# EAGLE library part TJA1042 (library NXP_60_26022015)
High-speed CAN transceiver with Standby mode The TJA1042 is a high-speed CAN transceiver that provides an interface between a Controller Area Network (CAN) protocol controller and the physical two-wire CAN bus. The transceiver is designed for high-speed (up to 1 Mbit/s) CAN applications in the automotive industry, providing the differential transmit and receive capability to (a microcontroller with) a CAN protocol controller. The TJA1042 belongs to the third generation of high-speed CAN transceivers from NXP Semiconductors, offering significant improvements over first- and second-generation devices such as the TJA1040. It offers improved ElectroMagnetic Compatibility (EMC) and ElectroStatic Discharge (ESD) performance, and also features: Ideal passive behavior to the CAN bus when the supply voltage is off A very low-current Standby mode with bus wake-up capability TJA1042T/3 and TJA1042TK/3 can be interfaced directly to microcontrollers with supply voltages from 3 V to 5 V These features make the TJA1042 an excellent choice for all types of HS-CAN networks, in nodes that require a low-power mode with wake-up capability via the CAN bus. AAL Eindhoven MK
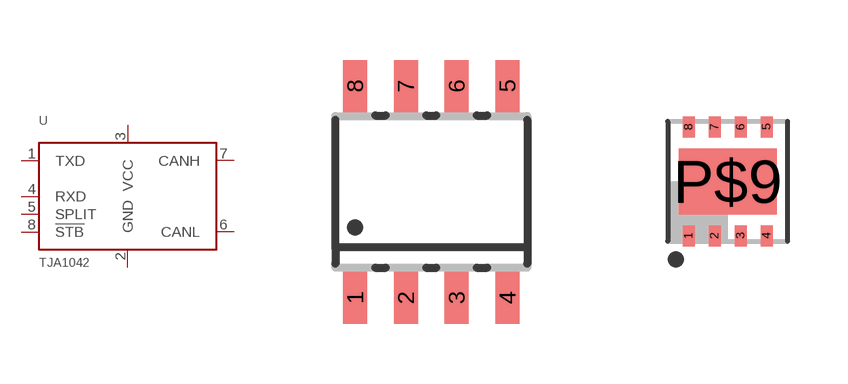
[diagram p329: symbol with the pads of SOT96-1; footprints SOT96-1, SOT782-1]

Designator prefix U

## TJA1042T  [SOT96-1]
1  TXD  out
2  GND  pwr
3  VCC  pwr
4  RXD
5  SPLIT  pwr
6  CANL
7  CANH
8  !STB  in

## TJA1042TK  [SOT782-1]
Pads as for SOT96-1

## Footprint SOT96-1 (pad centres in mm)
SOT96-1 SO8: plastic small outline package; 8 leads; body width 3.9 mm JEDEC: MS-012 IEC: 076E03
smd 0.6 x 1.3: 1 -1.905,-2.65; 2 -0.635,-2.65; 3 0.635,-2.65; 4 1.905,-2.65; 5 1.905,2.65; 6 0.635,2.65; 7 -0.635,2.65; 8 -1.905,2.65

## Footprint SOT782-1 (pad centres in mm)
SOT782-1 HVSON8: plastic thermal enhanced very thin small outline package; no leads; 8 terminals; body 3 x 3 x 0.85 mm JEDEC: MO-229 IEC: -- JEITA: --
smd 0.3 x 0.525: 1 -0.975,-1.363; 2 -0.325,-1.363; 3 0.325,-1.363; 4 0.975,-1.363; 5 0.975,1.363; 6 0.325,1.363; 7 -0.325,1.363; 8 -0.975,1.363
smd 2.45 x 1.65: P$9 0,0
